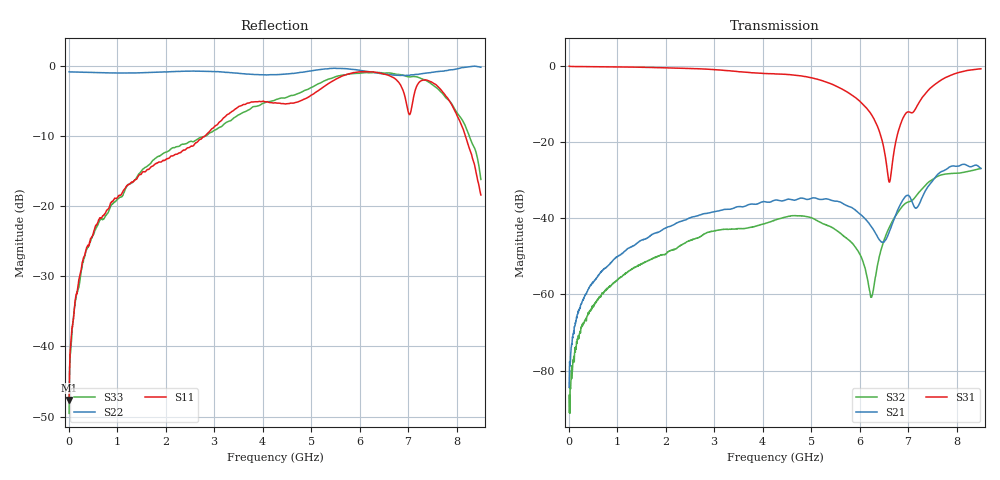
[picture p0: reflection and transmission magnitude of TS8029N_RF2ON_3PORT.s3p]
!Created with skrf (http://scikit-rf.org).
# GHz S RI R 50.0
!freq ReS11 ImS11 ReS12 ImS12 ReS13 ImS13
! ReS21 ImS21 ReS22 ImS22 ReS23 ImS23
! ReS31 ImS31 ReS32 ImS32 ReS33 ImS33
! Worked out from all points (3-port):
!   1601 points, 10 MHz to 8.5 GHz, reference 50 ohm
!   strongest paths, dB at 10 MHz, 2.132 GHz, 4.255 GHz, 6.378 GHz, 8.5 GHz:
!     S31: -0.1, -0.5, -2.1, -16.2, -0.8
!     S21: -84.4, -41.9, -35.2, -45.1, -26.9
!     S32: -91.0, -48.3, -40.5, -51.8, -26.9
!   lowest |S11| = -47.6 dB at 10 MHz (marker M1), VSWR 1.01, Z = 50.1 + j0.392 ohm
!   |S11| at or under -10 dB: start of sweep to 2.816 GHz; 8.178 GHz to end of sweep
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0.01  0.0014 0.00391  -9.49e-07 7.37e-05  0.9932 -0.00913
      -2.88e-06 6e-05  -0.9048 0.00338  3.71e-06 1.25e-05
      0.9932 -0.00917  1.23e-05 2.55e-05  0.00279 0.00183
0.3177625  0.00687 -0.0431  1.68e-05 0.00091  0.9736 -0.1146
           2.58e-05 0.000908  -0.8942 0.0762  -8.97e-05 -0.000407
           0.9737 -0.1147  -8.32e-05 -0.000422  0.00214 -0.0425
0.9704312  -0.0301 -0.1093  -0.000312 0.00302  0.9102 -0.3373
           -0.00032 0.00304  -0.8535 0.2447  -0.0013 -0.000762
           0.9103 -0.3372  -0.00131 -0.000737  -0.0251 -0.1049
4.255  -0.5438 0.0194  0.00842 0.0151  -0.06 -0.7852
       0.00841 0.0151  -0.3394 0.7942  -0.000505 0.00945
       -0.0613 -0.7837  -0.000466 0.00946  -0.5678 -0.0213
5.581563  -0.577 0.5881  0.0137 0.00912  -0.3499 -0.3826
          0.0138 0.00913  -0.0392 0.9561  0.00475 0.00442
          -0.3499 -0.382  0.00476 0.0044  -0.5842 0.6147
6.244844  -0.2405 0.87  0.00635 0.00435  -0.2051 -0.1011
          0.00637 0.00435  -0.00393 0.9017  -0.000283 0.00091
          -0.2054 -0.1009  -0.000285 0.000872  -0.4176 0.7863
6.610975  0.0455 0.8481  -0.00193 0.00632  -0.00344 -0.0295
          -0.00191 0.00633  0.1012 0.8584  -0.00734 0.00193
          -0.00347 -0.0296  -0.00733 0.00196  -0.0349 0.886
6.950575  0.2765 0.497  -0.00272 0.0192  0.1705 -0.1648
          -0.00272 0.0193  0.2565 0.8111  -0.012 0.0103
          0.1709 -0.165  -0.0119 0.0103  0.3733 0.7541
7.709369  0.5454 0.3571  0.000766 0.0414  0.2649 -0.6132
          0.000852 0.0414  0.4925 0.768  -0.00101 0.0374
          0.2643 -0.6152  -0.00109 0.0374  0.532 0.3435
8.5  0.0766 0.0923  0.0233 0.0385  -0.2253 -0.8885
     0.0234 0.0385  0.4947 0.8403  0.018 0.0415
     -0.2264 -0.8885  0.0179 0.0414  0.1527 0.0257
